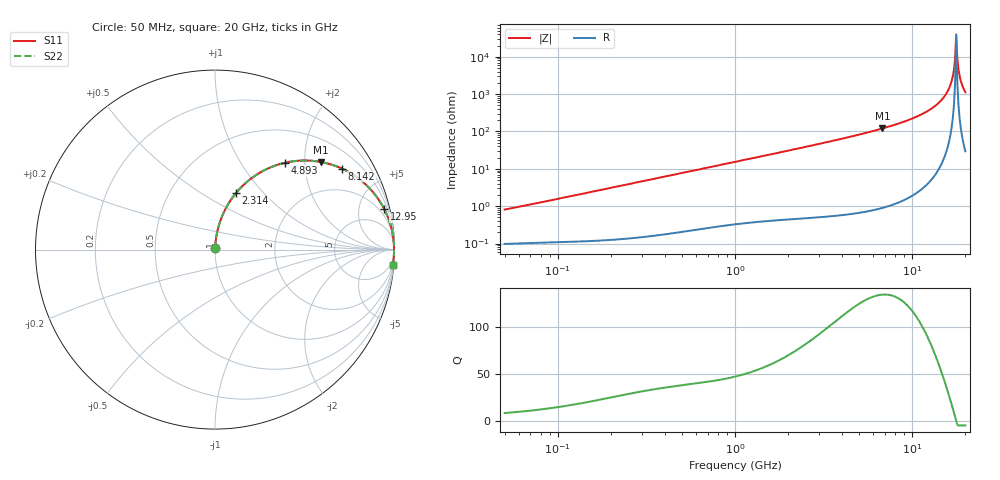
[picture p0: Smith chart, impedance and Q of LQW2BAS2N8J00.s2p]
!Murata Part Number: LQW2BAS2N8J00
!These Parameters are Measured in Series Mode Connection
!  o--[Z]--o
!Port1  Port2
!  o-------o
!Freq. Start=50[MHz] Stop=20[GHz], 401[Steps]
# Hz S RI R 50
!Freq.(Hz) S11(Real) S11(Imag) S21(Real) S21(Imag) S12(Real) S12(Imag) S22(Real) S22(Imag)
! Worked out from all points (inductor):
!   401 points, 50 MHz to 20 GHz, reference 50 ohm
!   read as one part in series: L = 2.53 nH near 51.52 MHz
!   highest Q = 134 at 6.802 GHz (marker M1), where L = 2.82 nH
!   self-resonance near 17.74 GHz
!   S11 on the Smith chart (normalised r, x): 50 MHz: 1.00, +0.02; 2.314 GHz: 1.01, +0.71; 4.893 GHz: 1.01, +1.60; 8.142 GHz: 1.02, +3.12; 12.95 GHz: 1.11, +8.38; 20 GHz: 2, -22
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5e7  0.00104 0.00802  0.999 -0.00802  0.999 -0.00802  0.00104 0.00802
1.364002e8  0.00159 0.0213  0.9984 -0.0213  0.9984 -0.0213  0.00159 0.0213
3.721004e8  0.00498 0.0573  0.995 -0.0573  0.995 -0.0573  0.00498 0.0573
1e9  0.026 0.149  0.974 -0.149  0.974 -0.149  0.026 0.149
2.313601e9  0.1162 0.3141  0.8838 -0.3141  0.8838 -0.3141  0.1162 0.3141
2.728004e9  0.1549 0.3561  0.8451 -0.3561  0.8451 -0.3561  0.1549 0.3561
4.89267e9  0.3918 0.4841  0.6082 -0.4841  0.6082 -0.4841  0.3918 0.4841
6.802353e9  0.5919 0.4878  0.4081 -0.4878  0.4081 -0.4878  0.5919 0.4878
7.442007e9  0.6499 0.4733  0.3501 -0.4733  0.3501 -0.4733  0.6499 0.4733
8.141811e9  0.7071 0.4513  0.2929 -0.4513  0.2929 -0.4513  0.7071 0.4513
1.066139e10  0.8618 0.3405  0.1382 -0.3405  0.1382 -0.3405  0.8618 0.3405
1.295331e10  0.9435 0.2246  0.0565 -0.2246  0.0565 -0.2246  0.9435 0.2246
1.460232e10  0.9764 0.1426  0.0236 -0.1426  0.0236 -0.1426  0.9764 0.1426
1.597544e10  0.9913 0.0779  0.00874 -0.0779  0.00874 -0.0779  0.9913 0.0779
1.670968e10  0.9954 0.0448  0.00457 -0.0448  0.00457 -0.0448  0.9954 0.0448
1.696185e10  0.9963 0.0338  0.00368 -0.0338  0.00368 -0.0338  0.9963 0.0338
1.721783e10  0.997 0.0227  0.00303 -0.0227  0.00303 -0.0227  0.997 0.0227
1.774144e10  0.9975 0.00048  0.00247 -0.00048  0.00247 -0.00048  0.9975 0.00048
1.828096e10  0.9971 -0.0217  0.00291 0.0217  0.00291 0.0217  0.9971 -0.0217
1.855685e10  0.9965 -0.0328  0.0035 0.0328  0.0035 0.0328  0.9965 -0.0328
1.912117e10  0.9946 -0.0549  0.00542 0.0549  0.00542 0.0549  0.9946 -0.0549
2e10  0.9899 -0.0879  0.0101 0.0879  0.0101 0.0879  0.9899 -0.0879
